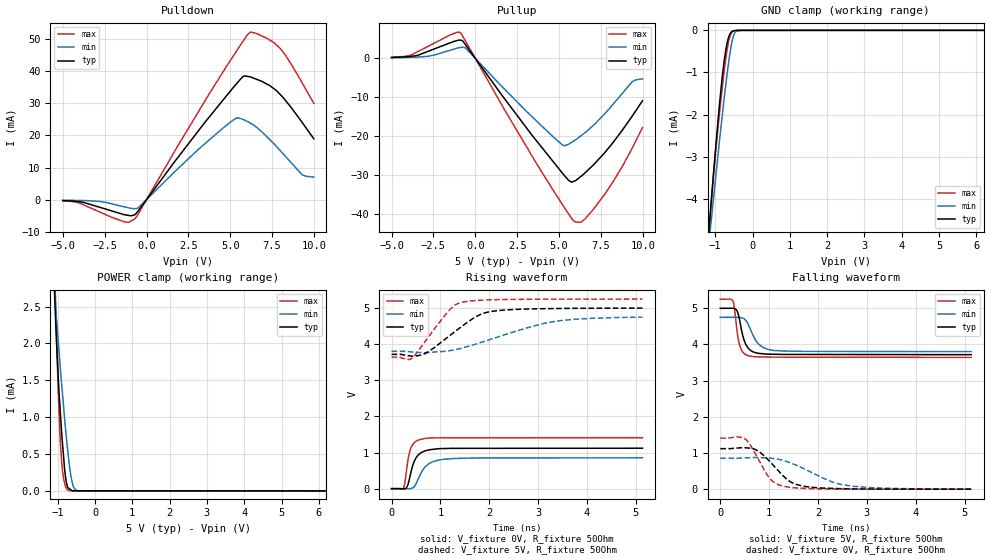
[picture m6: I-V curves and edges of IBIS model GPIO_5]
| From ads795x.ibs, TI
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|   Output GPIO model 5V
[Model]   GPIO_5
Model_type   I/O
|Signals   GPIO0, GPIO1, GPIO2, GPIO3
| variable   typ   min   max
Vinl = 0.8
Vinh = 3.5
Vmeas = 2.5
Vref = 2.5
Cref = 15pF
Rref = 50
|   typ   min   max
|C_comp Input mode
C_comp   1.0139468e-12   1.2214638e-12   8.1230338e-13
|C_comp Output High
|C_comp   1.9453807e-10   1.0043666e-10   3.2713408e-10
|C_comp Output Low
|C_comp   1.1350961e-10   6.1681443e-11   2.0681106e-10
[Voltage Range]   5   4.75   5.25
[Temperature Range]   27   125   -40
[Pullup Reference]   5   4.75   5.25
[Pulldown Reference]   0   0   0
[Power Clamp Reference]   5   4.75   5.25
[GND Clamp Reference]   0   -0   0
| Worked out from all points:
|   slope of the pulldown table from 0 to 0.75 V, typ, clamps not added: 142 ohm
|   slope of the pullup table from 0 to 0.75 V, typ, clamps not added: 168 ohm
|   GND clamp passes 1 mA (typ) near -0.80 V on its own axis
|   POWER clamp passes 1 mA (typ) near -0.92 V on its own axis
|   falling waveform, V_fixture 5V, R_fixture 50Ohm: 20-80 % time 151ps typ, 230ps min, 104ps max; typ from 5 V to 3.72 V
|   rising waveform, V_fixture 0V, R_fixture 50Ohm: 20-80 % time 166ps typ, 247ps min, 113ps max; typ from 0 V to 1.12 V
|   rising waveform, V_fixture 5V, R_fixture 50Ohm: 20-80 % time 765ps typ, 1.38ns min, 546ps max; typ from 3.72 V to 5 V
|   falling waveform, V_fixture 0V, R_fixture 50Ohm: 20-80 % time 495ps typ, 837ps min, 367ps max; typ from 1.12 V to 0 V
[Pulldown]
|   Voltage   I(typ)   I(min)   I(max)
-5V       -320uA     -173.3uA   -370.5uA
-4.04V    -653.3uA   -265.8uA   -1mA
-1.321V   -4.704mA   -2.263mA   -6.967mA
-709.3mV  -4.755mA   -2.848mA   -5.993mA
-466.4mV  -3.275mA   -2.434mA   -4.184mA
5.241V    35.33mA    25.07mA    45.28mA
5.829V    38.57mA    24.83mA    49.91mA
6.181V    38.28mA    23.92mA    52.21mA
7.155V    36.12mA    19.75mA    50.39mA
7.978V    32.81mA    15.32mA    47.18mA
9.292V    24.07mA    7.756mA    36.43mA
9.985V    18.99mA    7.033mA    30.03mA
[GND Clamp]
|   Voltage   I(typ)   I(min)   I(max)
-5V       -49.83mA   -40.16mA   -61.95mA
-1.164V   -4.683mA   -5.009mA   -4.811mA
-1.105V   -4.036mA   -4.501mA   -4.102mA
-1.013V   -3.055mA   -3.706mA   -3.128mA
-895.2mV  -1.854mA   -2.707mA   -2.055mA
-766.7mV  -774.5uA   -1.666mA   -1.019mA
-707.8mV  -424.8uA   -1.227mA   -614.6uA
-635.2mV  -152.2uA   -729.8uA   -242.5uA
-557.7mV  -31.96uA   -300.8uA   -51.54uA
-504.5mV  -8.613uA   -118.8uA   -12.03uA
-299.4mV  -691.6nA   -478.1nA   -752.1nA
9.985V    0A         0A         0A
[Pullup]
|   Voltage   I(typ)   I(min)   I(max)
-5V       232.9uA    156.6uA    284.4uA
-3.849V   500uA      261.2uA    827.1uA
-896.2mV  4.66mA     2.781mA    6.586mA
-550.6mV  3.29mA     2.519mA    4.165mA
1.721V    -10.18mA   -7.772mA   -12.97mA
5.176V    -29.26mA   -22.09mA   -37.25mA
5.739V    -31.7mA    -21.56mA   -40.88mA
6.012V    -31.25mA   -20.81mA   -41.96mA
6.528V    -29.44mA   -19.12mA   -41.26mA
7.733V    -24.15mA   -14.17mA   -34.8mA
9.381V    -14.75mA   -5.948mA   -22.94mA
9.985V    -10.87mA   -5.255mA   -17.75mA
[POWER Clamp]
|   Voltage   I(typ)   I(min)   I(max)
-5V       75.77mA    59.83mA    93.41mA
-1.081V   2.634mA    2.699mA    3.001mA
-1.068V   2.46mA     2.597mA    2.759mA
-1.05V    2.232mA    2.454mA    2.416mA
-975.3mV  1.432mA    1.959mA    1.198mA
-937.7mV  1.12mA     1.71mA     745.7uA
-896.2mV  793.3uA    1.456mA    406.3uA
-788.6mV  180.9uA    826.1uA    53.31uA
-659.7mV  19.98uA    245.1uA    1.163uA
-572.5mV  964.8nA    48.38uA    1.153uA
-431.9mV  952nA      1.07uA     1.138uA
9.985V    0A         0A         0A
[Ramp]
R_load = 50
|   typ   min   max
dV/dt_r   0.672068/1.65249e-010  0.512528/2.43736e-010  0.846699/1.1289e-010
dV/dt_f   0.768929/1.49038e-010  0.568592/2.27547e-010  0.963985/1.04184e-010
[Falling Waveform]
V_fixture = 5V
V_fixture_min = 4.75V
V_fixture_max = 5.25V
R_fixture = 50Ohm
C_fixture = 0F
|   Time   V(typ)   V(min)   V(max)
0s        5V         4.75V      5.25V
257.9ps   5.002V     4.75V      5.202V
289.6ps   4.992V     4.75V      4.996V
344.9ps   4.927V     4.75V      4.351V
397.5ps   4.656V     4.747V     3.976V
488.2ps   4.115V     4.709V     3.752V
588ps     3.877V     4.507V     3.683V
782.7ps   3.754V     4.012V     3.656V
1.096ns   3.73V      3.835V     3.651V
5.135ns   3.718V     3.802V     3.643V
[Rising Waveform]
V_fixture = 0V
V_fixture_min = 0V
V_fixture_max = 0V
R_fixture = 50Ohm
C_fixture = 0F
|   Time   V(typ)   V(min)   V(max)
0s        -441.3nV   -422.4nV   -433.7nV
240.4ps   -6.61mV    -2.21mV    18.87mV
272.1ps   -2.017mV   -2.501mV   169.8mV
323.8ps   68.38mV    -2.976mV   684.9mV
399.4ps   467mV      4.184mV    1.135V
504.7ps   861.7mV    149.3mV    1.316V
673.3ps   1.04V      578.8mV    1.389V
859.2ps   1.09V      753mV      1.405V
1.307ns   1.116V     837.7mV    1.408V
5.135ns   1.12V      854.2mV    1.411V
[Rising Waveform]
V_fixture = 5V
V_fixture_min = 4.75V
V_fixture_max = 5.25V
R_fixture = 50Ohm
C_fixture = 0F
|   Time   V(typ)   V(min)   V(max)
0s        3.718V     3.802V     3.643V
354.8ps   3.68V      3.793V     3.573V
420.6ps   3.67V      3.784V     3.618V
676ps     3.736V     3.763V     4.054V
1.168ns   4.213V     3.818V     4.92V
1.431ns   4.488V     3.889V     5.159V
1.829ns   4.83V      4.049V     5.218V
2.173ns   4.93V      4.199V     5.234V
3.408ns   4.989V     4.644V     5.248V
5.135ns   5V         4.75V      5.25V
[Falling Waveform]
|Gnd
V_fixture = 0V
V_fixture_min = 0V
V_fixture_max = 0V
R_fixture = 50Ohm
C_fixture = 0F
|   Time   V(typ)   V(min)   V(max)
0s        1.12V      854.2mV    1.411V
502.7ps   1.146V     865mV      1.394V
730.5ps   1.087V     878.1mV    949.2mV
1.014ns   763.7mV    860.2mV    293.7mV
1.319ns   327.3mV    781.4mV    73.86mV
1.462ns   183.8mV    712.8mV    44.86mV
1.734ns   75.88mV    551.3mV    21.81mV
2.295ns   21.43mV    197.6mV    4.491mV
2.674ns   7.978mV    86.55mV    1.767mV
5.135ns   -441.3nV   -422.4nV   -433.7nV
